(* Logix 5000 AddOnInstructionDefinition export EH_Promass10_IOL; software revision 38.00 *)

TYPE EH_CommAOI_Data :
STRUCT
   Device_Comm_Error : BOOL;
   CommSuccess : BOOL;
   CommFailed : BOOL;
   CommTimeOut : BOOL;
   StateDone : BOOL;
   NewState : BOOL;
   OldState : SINT;
   PortSize : SINT;
   DevicePort : SINT;
   MaxState : SINT;
   State : SINT;
   VendorID : INT;
   DeviceID : DINT;
   CyclicData : INT[16];
   AcyclicData : DINT[8];
   ReplayIndex : INT;
   AOI_Diagnostic : DINT;
   ConnectionStatus : DINT;
   OutputData : INT[16];
END_STRUCT
END_TYPE

ADD_ON_INSTRUCTION EH_Promass10_IOL   (* revision 1.2, vendor Endress+Hauser *)
// Promass 10 Rev 1 IO-Link
// Revision note:
// 1.2 Added HeartbeatVerification
// 1.1 Changed the Datatype from Unsigned to Signed
// Add Disconnect check
VAR_IN_OUT
   DataToSend : INT[10]; {required}
   CommAOIBusy : DINT; {required}
   ActiveComPort : DINT; {required}
   DeviceAOISendRequest : DINT; {required}
   CommError : INT; {required}
   DeviceData : EH_CommAOI_Data; {required}
END_VAR
VAR_INPUT
   iSetSimulation : BOOL; {visible}
   iSimulationVariable : INT; {visible}
   iSimulationValue : REAL; {visible}
   iSetTotalizerPresetValue : BOOL; {visible}
   iTotalizerPresetValue : REAL; {visible}
   iTotalizer_Hold : BOOL; {visible}
   iTotalizer_ResetTotalize : BOOL; {visible}
   iTotalizer_ResetHold : BOOL; {visible}
   iTotalizer_Totalize : BOOL; {visible}
   iDeviceSearch : BOOL; {visible}
   iFlowOverride : BOOL; {visible}
   iStart_HeartbeatVerification : BOOL; {visible}
END_VAR
VAR_OUTPUT
   qVendor_ID : DINT; {access Read Only, visible}
   qDevice_ID : DINT; {access Read Only, visible}
   qMassFlow : REAL; {access Read Only, visible}
   qDensity : REAL; {access Read Only, visible}
   qTemperature : REAL; {visible}
   qTotalizer1 : REAL; {access Read Only, visible}
   qExtendedDeviceStatus : INT; {access Read Only, visible}
   qSSC1_1 : BOOL; {access Read Only, visible}
   qSSC1_2 : BOOL; {access Read Only, visible}
   qSSC2_1 : BOOL; {access Read Only, visible}
   qSSC2_2 : BOOL; {access Read Only, visible}
   qSSC3_1 : BOOL; {access Read Only, visible}
   qSSC3_2 : BOOL; {access Read Only, visible}
   qSSC4_1 : BOOL; {access Read Only, visible}
   qSSC4_2 : BOOL; {access Read Only, visible}
   qProgress : SINT; {visible}
   qVerificationID : INT; {visible}
   qPassed : BOOL; {access None, visible}
   qFailed : BOOL; {access None, visible}
   qAOI_Diagnostic : DINT; {access Read Only, visible}
END_VAR
VAR_IN_OUT
   qAOI_Diagnostic_String : STRING; {required}
END_VAR
VAR_OUTPUT
   qActual_Diagnostics_Code : DINT; {access Read Only, visible}
END_VAR
VAR_IN_OUT
   qActual_Diagnostics_String : STRING; {required}
END_VAR
VAR_OUTPUT
   qLast_Diagnostics_Code : DINT; {visible}
END_VAR
VAR_IN_OUT
   qLast_Diagnostics_String : STRING; {required}
END_VAR
VAR_OUTPUT
   qCommError : DINT; {access None}
   qCommunicationBusy : DINT; {access Read Only, visible}
   qDeviceConnectionError : BOOL; {access Read Only, visible}
END_VAR
VAR
   Calc_DID : DINT; {access None}
   Calc_VID : DINT; {access None}
   Calc_Data : DINT; {access None}
   Cond_DINT : DINT; {access None}
   Temp_DINT : DINT; {access None}
   Calc_Cond : DINT; {access None}
   Cald_Temp : DINT; {access None}
   Calc_Temp : DINT; {access None}
   Calc_CondenStatus : DINT; {access None}
   CMD_Index : INT; {access None}
   CMD_Subindex : INT; {access None}
   CMD_ByteLength : INT; {access None}
   oldCondStatus : INT; {access None}
   SetSimulation : SINT; {access None}
   SetTotalizer : SINT; {access None}
   oldSetSimulation : SINT; {access None}
   oldSetTotalizer : SINT; {access None}
   Trigger : BOOL; {access None}
   CMD_Rd : BOOL; {access None}
   CMD_Wr : BOOL; {access None}
   SimulationDINT : DINT; {access None}
   SimulationReal : DINT; {access None}
   Calc_Out : DINT; {access None}
   Calc_Level : DINT; {access None}
   Calc_Pressure : DINT; {access None}
   Pressure_DINT : DINT; {access None}
   Level_DINT : DINT; {access None}
   InputByteLength : DINT; {access None}
   AOI_Prio : BOOL; {access None}
   ActiveAOI : BOOL; {access None}
   StateMin : DINT; {access None}
   firstTimeDone : BOOL; {access None}
   Calc_Connection_Status : DINT; {access None}
   NextStep : BOOL; {access None}
   OldStatus : DINT; {access None}
   ChangedStatus : BOOL; {access None}
   CondStatusChanged : BOOL; {access None}
   Calc_MassFlow : DINT; {access None}
   Calc_Density : DINT; {access None}
   Calc_Temperature : DINT; {access None}
   Calc_Totalizer1 : DINT; {access None}
   Calc_ExtendedDeviceStatus : DINT; {access None}
   MassFlow_DINT : DINT; {access None}
   Density_DINT : DINT; {access None}
   Totalizer1_DINT : DINT; {access None}
   SimChanged : BOOL; {access None}
   TotChanged : BOOL; {access None}
   Skip : BOOL; {access None}
   CondStatusActive : BOOL; {access None}
   SimActive : BOOL; {access None}
   TotActive : BOOL; {access None}
   DeviceID : DINT; {access None}
   FALSE : BOOL; {access None}
   TRUE : BOOL := 1; {access None}
   temp_string1 : STRING; {access None}
   temp_string2 : STRING; {access None}
   Start_HeartbeatVerification : SINT; {access None}
   oldStart_HeartbeatVerification : SINT; {access None}
   HeartbeatVerificationChanged : BOOL; {access None}
   HeartbeatVerificationActive : BOOL; {access None}
END_VAR

ROUTINE Logic   (* structured text *)
// Picomag Communication via AL1323
   // =======================================================================
   // Endress+Hauser Digital Solutions
   // ©Copyright (2024) All Rights Reserved
   // =======================================================================
   // Name:                EH_Promass10_IOL
   // Version:             1.2
   // Datum:               11.2025
   // Library:             01.01.00
   // Engineering:         Studio5000 V38.00.00
   // Author:              EH
   // =======================================================================
   
   qAOI_Diagnostic := DeviceData.AOI_Diagnostic;
   qCommunicationBusy := CommAOIBusy;
   DeviceID := 9728513;
   StateMin := 0;
   DeviceData.MaxState := 98;
   
   if DeviceData.DevicePort = 0 or DeviceData.DeviceID <> DeviceID or DeviceData.ConnectionStatus <> 1 then
   
   	qVendor_ID := DeviceData.VendorID;
   	qDevice_ID := DeviceData.DeviceID;
   	qMassFlow	:= 0;
   	qDensity	:= 0;
   	qTemperature	:= 0;
   	qTotalizer1	:= 0;
   	qExtendedDeviceStatus	:= 0;
   	qSSC1_1	:= 0;
   	qSSC1_2	:= 0;
   	qSSC2_1	:= 0;
   	qSSC2_2	:= 0;
   	qSSC3_1	:= 0;
   	qSSC3_2	:= 0;
   	qSSC4_1	:= 0;
   	qSSC4_2	:= 0;
   	qActual_Diagnostics_Code	:= 0;
   	qLast_Diagnostics_Code	:= 0;
   	qLast_Diagnostics_String	:= '';
   	qPassed := FALSE;
   	qFailed := FALSE;
   	oldCondStatus := 0;
   	CondStatusChanged := FALSE;
   
   	if DeviceData.DevicePort = 0 then
   
   		qActual_Diagnostics_String	:= 'Device Port is Zero';
   		DeviceData.AOI_Diagnostic.1 := TRUE;
   
   	elsif DeviceData.ConnectionStatus <> 1 then
   
   		qActual_Diagnostics_String	:= 'No Device connected';
   		qDeviceConnectionError := TRUE;
   
   	elsif DeviceData.DeviceID <> DeviceID then
   
   		qActual_Diagnostics_String	:= 'Wrong DeviceID';
   		DeviceData.AOI_Diagnostic.2 := TRUE;
   	end_if;
   
   else
   
   	if qActual_Diagnostics_Code = 0  then
   
   		qActual_Diagnostics_String	:= '--------';
   
   	end_if;
   
   	if qLast_Diagnostics_Code = 0 then
   
   		qLast_Diagnostics_String	:= '--------';
   
   	end_if;
   
   	DeviceData.AOI_Diagnostic.1 := FALSE;
   	qDeviceConnectionError := FALSE;
   	DeviceData.AOI_Diagnostic.2  := FALSE;
   
   end_if;
   
   // Case device disconnected during communication to avoid blocking the communication
   if (DeviceData.AOI_Diagnostic.0 or qDeviceConnectionError or DeviceData.AOI_Diagnostic.2) and ActiveAOI and ActiveComPort = DeviceData.DevicePort and CommAOIBusy = 1 then
   
   	DeviceData.State := 0;
   	CommAOIBusy := 0;
   	DeviceAOISendRequest.[DeviceData.DevicePort] := 0;
   	ActiveComPort := 0;
   	ActiveAOI := 0;
   	DataToSend[0] := 0;
   	DataToSend[1] := 0;
   	DataToSend[2] := 0;
   	DataToSend[3] := 0;
   	DataToSend[4] := 0;
   	DataToSend[5] := 0;
   	DataToSend[6] := 0;
   	DataToSend[7] := 0;
   	DataToSend[8] := 0;
   	DataToSend[9] := 0;
   	DeviceData.StateDone := FALSE;
   	DeviceData.NewState := FALSE;
   	DeviceData.OldState := 0;
   	ActiveAOI := FALSE;
   
   end_if;
   
   if not DeviceData.AOI_Diagnostic.0
   	and not qDeviceConnectionError
   	and not DeviceData.AOI_Diagnostic.2
   	and DeviceData.DevicePort > 0 then
   
   	//*********************************
   	//Vendor ID
   	//*********************************
   
   		qVendor_ID := DeviceData.VendorID;
   
   	//*********************************
   	//Device ID
   	//*********************************
   
   		qDevice_ID := DeviceData.DeviceID;
   
   	//*********************************
   	// Promag 10 Cyclic Input
   	//*********************************
   
   		Calc_MassFlow				:= 0;
   		Calc_Density				:= 2;
   		Calc_Temperature			:= 4;
   		Calc_Totalizer1				:= 6;
   		Calc_ExtendedDeviceStatus	:= 8;
   
   	//*********************************
   	//Process Data MassFlow
   	//*********************************
   
   		Temp_DINT	 := DeviceData.CyclicData[Calc_MassFlow+1];
   		Temp_DINT.8	 := DeviceData.CyclicData[Calc_MassFlow+1].8;
   		Temp_DINT.9  := DeviceData.CyclicData[Calc_MassFlow+1].9;
   		Temp_DINT.10 := DeviceData.CyclicData[Calc_MassFlow+1].10;
   		Temp_DINT.11 := DeviceData.CyclicData[Calc_MassFlow+1].11;
   		Temp_DINT.12 := DeviceData.CyclicData[Calc_MassFlow+1].12;
   		Temp_DINT.13 := DeviceData.CyclicData[Calc_MassFlow+1].13;
   		Temp_DINT.14 := DeviceData.CyclicData[Calc_MassFlow+1].14;
   		Temp_DINT.15 := DeviceData.CyclicData[Calc_MassFlow+1].15;
   		Temp_DINT.16 := DeviceData.CyclicData[Calc_MassFlow].0;
   		Temp_DINT.17 := DeviceData.CyclicData[Calc_MassFlow].1;
   		Temp_DINT.18 := DeviceData.CyclicData[Calc_MassFlow].2;
   		Temp_DINT.19 := DeviceData.CyclicData[Calc_MassFlow].3;
   		Temp_DINT.20 := DeviceData.CyclicData[Calc_MassFlow].4;
   		Temp_DINT.21 := DeviceData.CyclicData[Calc_MassFlow].5;
   		Temp_DINT.22 := DeviceData.CyclicData[Calc_MassFlow].6;
   		Temp_DINT.23 := DeviceData.CyclicData[Calc_MassFlow].7;
   		Temp_DINT.24 := DeviceData.CyclicData[Calc_MassFlow].8;
   		Temp_DINT.25 := DeviceData.CyclicData[Calc_MassFlow].9;
   		Temp_DINT.26 := DeviceData.CyclicData[Calc_MassFlow].10;
   		Temp_DINT.27 := DeviceData.CyclicData[Calc_MassFlow].11;
   		Temp_DINT.28 := DeviceData.CyclicData[Calc_MassFlow].12;
   		Temp_DINT.29 := DeviceData.CyclicData[Calc_MassFlow].13;
   		Temp_DINT.30 := DeviceData.CyclicData[Calc_MassFlow].14;
   		Temp_DINT.31 := DeviceData.CyclicData[Calc_MassFlow].15;
   
   		COP(Temp_DINT,qMassFlow,1);
   
   	//*********************************
   	//Process Data Density
   	//*********************************
   
   		Temp_DINT	 := DeviceData.CyclicData[Calc_Density+1];
   		Temp_DINT.8	 := DeviceData.CyclicData[Calc_Density+1].8;
   		Temp_DINT.9	 := DeviceData.CyclicData[Calc_Density+1].9;
   		Temp_DINT.10 := DeviceData.CyclicData[Calc_Density+1].10;
   		Temp_DINT.11 := DeviceData.CyclicData[Calc_Density+1].11;
   		Temp_DINT.12 := DeviceData.CyclicData[Calc_Density+1].12;
   		Temp_DINT.13 := DeviceData.CyclicData[Calc_Density+1].13;
   		Temp_DINT.14 := DeviceData.CyclicData[Calc_Density+1].14;
   		Temp_DINT.15 := DeviceData.CyclicData[Calc_Density+1].15;
   		Temp_DINT.16 := DeviceData.CyclicData[Calc_Density].0;
   		Temp_DINT.17 := DeviceData.CyclicData[Calc_Density].1;
   		Temp_DINT.18 := DeviceData.CyclicData[Calc_Density].2;
   		Temp_DINT.19 := DeviceData.CyclicData[Calc_Density].3;
   		Temp_DINT.20 := DeviceData.CyclicData[Calc_Density].4;
   		Temp_DINT.21 := DeviceData.CyclicData[Calc_Density].5;
   		Temp_DINT.22 := DeviceData.CyclicData[Calc_Density].6;
   		Temp_DINT.23 := DeviceData.CyclicData[Calc_Density].7;
   		Temp_DINT.24 := DeviceData.CyclicData[Calc_Density].8;
   		Temp_DINT.25 := DeviceData.CyclicData[Calc_Density].9;
   		Temp_DINT.26 := DeviceData.CyclicData[Calc_Density].10;
   		Temp_DINT.27 := DeviceData.CyclicData[Calc_Density].11;
   		Temp_DINT.28 := DeviceData.CyclicData[Calc_Density].12;
   		Temp_DINT.29 := DeviceData.CyclicData[Calc_Density].13;
   		Temp_DINT.30 := DeviceData.CyclicData[Calc_Density].14;
   		Temp_DINT.31 := DeviceData.CyclicData[Calc_Density].15;
   
   		COP(Temp_DINT,qDensity,1);
   
   	//*********************************
   	// Process Parameter Temperature
   	//*********************************
   
   		Temp_DINT	 := DeviceData.CyclicData[Calc_Temperature+1];
   		Temp_DINT.8	 := DeviceData.CyclicData[Calc_Temperature+1].8;
   		Temp_DINT.9	 := DeviceData.CyclicData[Calc_Temperature+1].9;
   		Temp_DINT.10 := DeviceData.CyclicData[Calc_Temperature+1].10;
   		Temp_DINT.11 := DeviceData.CyclicData[Calc_Temperature+1].11;
   		Temp_DINT.12 := DeviceData.CyclicData[Calc_Temperature+1].12;
   		Temp_DINT.13 := DeviceData.CyclicData[Calc_Temperature+1].13;
   		Temp_DINT.14 := DeviceData.CyclicData[Calc_Temperature+1].14;
   		Temp_DINT.15 := DeviceData.CyclicData[Calc_Temperature+1].15;
   		Temp_DINT.16 := DeviceData.CyclicData[Calc_Temperature].0;
   		Temp_DINT.17 := DeviceData.CyclicData[Calc_Temperature].1;
   		Temp_DINT.18 := DeviceData.CyclicData[Calc_Temperature].2;
   		Temp_DINT.19 := DeviceData.CyclicData[Calc_Temperature].3;
   		Temp_DINT.20 := DeviceData.CyclicData[Calc_Temperature].4;
   		Temp_DINT.21 := DeviceData.CyclicData[Calc_Temperature].5;
   		Temp_DINT.22 := DeviceData.CyclicData[Calc_Temperature].6;
   		Temp_DINT.23 := DeviceData.CyclicData[Calc_Temperature].7;
   		Temp_DINT.24 := DeviceData.CyclicData[Calc_Temperature].8;
   		Temp_DINT.25 := DeviceData.CyclicData[Calc_Temperature].9;
   		Temp_DINT.26 := DeviceData.CyclicData[Calc_Temperature].10;
   		Temp_DINT.27 := DeviceData.CyclicData[Calc_Temperature].11;
   		Temp_DINT.28 := DeviceData.CyclicData[Calc_Temperature].12;
   		Temp_DINT.29 := DeviceData.CyclicData[Calc_Temperature].13;
   		Temp_DINT.30 := DeviceData.CyclicData[Calc_Temperature].14;
   		Temp_DINT.31 := DeviceData.CyclicData[Calc_Temperature].15;
   
   		COP(Temp_DINT,qTemperature,1);
   
   	//*********************************
   	// Process Parameter Totalizer1
   	//*********************************
   
   		Temp_DINT	 := DeviceData.CyclicData[Calc_Totalizer1+1];
   		Temp_DINT.8	 := DeviceData.CyclicData[Calc_Totalizer1+1].8;
   		Temp_DINT.9	 := DeviceData.CyclicData[Calc_Totalizer1+1].9;
   		Temp_DINT.10 := DeviceData.CyclicData[Calc_Totalizer1+1].10;
   		Temp_DINT.11 := DeviceData.CyclicData[Calc_Totalizer1+1].11;
   		Temp_DINT.12 := DeviceData.CyclicData[Calc_Totalizer1+1].12;
   		Temp_DINT.13 := DeviceData.CyclicData[Calc_Totalizer1+1].13;
   		Temp_DINT.14 := DeviceData.CyclicData[Calc_Totalizer1+1].14;
   		Temp_DINT.15 := DeviceData.CyclicData[Calc_Totalizer1+1].15;
   		Temp_DINT.16 := DeviceData.CyclicData[Calc_Totalizer1].0;
   		Temp_DINT.17 := DeviceData.CyclicData[Calc_Totalizer1].1;
   		Temp_DINT.18 := DeviceData.CyclicData[Calc_Totalizer1].2;
   		Temp_DINT.19 := DeviceData.CyclicData[Calc_Totalizer1].3;
   		Temp_DINT.20 := DeviceData.CyclicData[Calc_Totalizer1].4;
   		Temp_DINT.21 := DeviceData.CyclicData[Calc_Totalizer1].5;
   		Temp_DINT.22 := DeviceData.CyclicData[Calc_Totalizer1].6;
   		Temp_DINT.23 := DeviceData.CyclicData[Calc_Totalizer1].7;
   		Temp_DINT.24 := DeviceData.CyclicData[Calc_Totalizer1].8;
   		Temp_DINT.25 := DeviceData.CyclicData[Calc_Totalizer1].9;
   		Temp_DINT.26 := DeviceData.CyclicData[Calc_Totalizer1].10;
   		Temp_DINT.27 := DeviceData.CyclicData[Calc_Totalizer1].11;
   		Temp_DINT.28 := DeviceData.CyclicData[Calc_Totalizer1].12;
   		Temp_DINT.29 := DeviceData.CyclicData[Calc_Totalizer1].13;
   		Temp_DINT.30 := DeviceData.CyclicData[Calc_Totalizer1].14;
   		Temp_DINT.31 := DeviceData.CyclicData[Calc_Totalizer1].15;
   
   		COP(Temp_DINT,qTotalizer1,1);
   
   	//*********************************
   	// Extended device Status
   	//*********************************
   
   		qExtendedDeviceStatus.0 := DeviceData.CyclicData[Calc_ExtendedDeviceStatus].8;
   		qExtendedDeviceStatus.1 := DeviceData.CyclicData[Calc_ExtendedDeviceStatus].9;
   		qExtendedDeviceStatus.2 := DeviceData.CyclicData[Calc_ExtendedDeviceStatus].10;
   		qExtendedDeviceStatus.3 := DeviceData.CyclicData[Calc_ExtendedDeviceStatus].11;
   		qExtendedDeviceStatus.4 := DeviceData.CyclicData[Calc_ExtendedDeviceStatus].12;
   		qExtendedDeviceStatus.5 := DeviceData.CyclicData[Calc_ExtendedDeviceStatus].13;
   		qExtendedDeviceStatus.6 := DeviceData.CyclicData[Calc_ExtendedDeviceStatus].14;
   		qExtendedDeviceStatus.7 := DeviceData.CyclicData[Calc_ExtendedDeviceStatus].15;
   
   	//*********************************
   	// Process Parameter SSC
   	//*********************************
   
   		qSSC1_1 := DeviceData.CyclicData[Calc_ExtendedDeviceStatus].0;
   		qSSC1_2 := DeviceData.CyclicData[Calc_ExtendedDeviceStatus].1;
   
   		qSSC2_1 := DeviceData.CyclicData[Calc_ExtendedDeviceStatus].2;
   		qSSC2_2 := DeviceData.CyclicData[Calc_ExtendedDeviceStatus].3;
   
   		qSSC3_1 := DeviceData.CyclicData[Calc_ExtendedDeviceStatus].4;
   		qSSC3_2 := DeviceData.CyclicData[Calc_ExtendedDeviceStatus].5;
   
   		qSSC4_1 := DeviceData.CyclicData[Calc_ExtendedDeviceStatus].6;
   		qSSC4_2 := DeviceData.CyclicData[Calc_ExtendedDeviceStatus].7;
   
   	//*********************************
   	// Process Output Parameter
   	//*********************************
   
   		DeviceData.OutputData[0].4 := iDeviceSearch;		//Device Specific
   		DeviceData.OutputData[0].5 := iFlowOverride;
   		DeviceData.OutputData[0].6 := iTotalizer_Hold;
   		DeviceData.OutputData[0].7 := iTotalizer_ResetTotalize;
   		DeviceData.OutputData[0].8 := iTotalizer_ResetHold;
   		DeviceData.OutputData[0].9 := iTotalizer_Totalize;
   
   	//*********************************
   	// Checking for Changed Status @ Input or Condenced Status
   	//*********************************
   
   	SetSimulation.0 := iSetSimulation;
   	SetTotalizer.0 := iSetTotalizerPresetValue;
   	Start_HeartbeatVerification.0 := iStart_HeartbeatVerification;
   
   	if oldCondStatus <> qExtendedDeviceStatus and not CondStatusChanged then
   
   		CondStatusChanged := TRUE;
   		oldCondStatus := qExtendedDeviceStatus;
   
   	end_if;
   
   	if oldSetSimulation <> SetSimulation and not SimChanged then
   
   		if oldSetSimulation < SetSimulation then
   
   			SimChanged := TRUE;
   
   		end_if;
   
   		oldSetSimulation := SetSimulation;
   
   	end_if;
   
   	if oldSetTotalizer <> SetTotalizer and not TotChanged then
   
   		if oldSetTotalizer < SetTotalizer then
   
   			TotChanged := TRUE;
   
   		end_if;
   
   		oldSetTotalizer := SetTotalizer;
   
   	end_if;
   
   	if oldStart_HeartbeatVerification <> Start_HeartbeatVerification and not HeartbeatVerificationChanged then
   
   		if oldStart_HeartbeatVerification < Start_HeartbeatVerification then
   
   			HeartbeatVerificationChanged := TRUE;
   
   		end_if;
   
   		oldStart_HeartbeatVerification := Start_HeartbeatVerification;
   
   	end_if;
   
   	if CondStatusChanged
   	and not ActiveAOI
   	and not CondStatusActive
   	and not Skip then
   
   		DeviceAOISendRequest.[DeviceData.DevicePort] := TRUE;
   		CondStatusActive := TRUE;
   		Skip := TRUE;
   
   	elsif SimChanged
   		and not ActiveAOI
   		and not SimActive
   		and not Skip then
   
   		DeviceAOISendRequest.[DeviceData.DevicePort] := TRUE;
   		SimActive := TRUE;
   		Skip := TRUE;
   
   	elsif TotChanged
   		and not ActiveAOI
   		and not TotActive
   		and not Skip then
   
   		DeviceAOISendRequest.[DeviceData.DevicePort] := TRUE;
   		TotActive := TRUE;
   		Skip := TRUE;
   
   	elsif HeartbeatVerificationChanged
   		and not ActiveAOI
   		and not HeartbeatVerificationActive
   		and not Skip then
   
   		DeviceAOISendRequest.[DeviceData.DevicePort] := TRUE;
   		HeartbeatVerificationActive := TRUE;
   		Skip := TRUE;
   
   	end_if;
   
   	if ActiveComPort = DeviceData.DevicePort then
   
   		AOI_Prio := TRUE;
   
   	else
   
   		AOI_Prio := FALSE;
   
   	end_if;
   
   	if (SimActive or TotActive or HeartbeatVerificationActive or CondStatusActive) and CommAOIBusy = 1  and DeviceData.State = 0 and AOI_Prio and not ActiveAOI then
   
   		ActiveAOI := TRUE;
   		Skip := FALSE;
   
   	end_if;
   
   	qCommunicationBusy := CommAOIBusy;
   	qAOI_Diagnostic :=DeviceData.AOI_Diagnostic;
   
   	//*********************************
   	// States for Execution
   	//*********************************
   
   	if ActiveAOI or DeviceData.State = DeviceData.MaxState then
   
   	case DeviceData.State of
   
   		//*********************************
   		0: // Start
   		//*********************************
   
   			Trigger := FALSE;
   			CMD_Index := 0;
   			CMD_Subindex := 0;
   			CMD_Wr := FALSE;
   			CMD_Rd := FALSE;
   			CMD_ByteLength := 0;
   
   			if DeviceData.DevicePort = ActiveComPort then
   
   				DeviceData.CommSuccess := FALSE;
   				DeviceData.CommTimeOut := FALSE;
   				DeviceData.NewState := TRUE;
   				DeviceData.StateDone := FALSE;
   
   			end_if;
   
   			if SimActive then
   
   				DeviceData.AOI_Diagnostic := 0;
   				DeviceData.State := 1;
   
   			elsif TotActive then
   				DeviceData.AOI_Diagnostic := 0;
   				DeviceData.State := 20;
   
   			elsif HeartbeatVerificationActive then
   
   				DeviceData.AOI_Diagnostic := 0;
   				DeviceData.State := 80;
   
   			elsif CondStatusChanged then
   
   				DeviceData.State := 90;
   
   			end_if;
   
   	//*********************************
   	1: // Set Simulation Variable
   	//*********************************
   
   			CMD_Index := 2066;
   			CMD_Subindex := 0;
   			CMD_Wr := TRUE;	// Only Read or Write can be active
   			CMD_Rd := FALSE;
   			CMD_ByteLength := 2;	//Check Length
   			DataToSend[6]:= 0;
   			DataToSend[7]:= 0;
   
   			// 0 = Off, 1 = Mass flow, 2 = Volume flow, 3 = Corrected volume flow, 4 = Density, 7 = Temperature
   			if iSimulationVariable > 0 then
   
   				DataToSend[6].8 := iSimulationVariable.0;
   				DataToSend[6].9 := iSimulationVariable.1;
   				DataToSend[6].10 := iSimulationVariable.2;
   				DataToSend[6].11 := iSimulationVariable.3;
   				DataToSend[6].12 := iSimulationVariable.4;
   				DataToSend[6].13 := iSimulationVariable.5;
   				DataToSend[6].14 := iSimulationVariable.6;
   				DataToSend[6].15 := iSimulationVariable.7;
   
   			else
   
   				DataToSend[6] := 0;
   				DataToSend[7] := 0;
   
   			end_if;
   
   			Trigger := TRUE;
   
   			if DeviceData.NewState then
   
   				DeviceData.StateDone := TRUE;
   
   			end_if;
   
   			if  DeviceData.CommSuccess and DeviceData.ReplayIndex = CMD_Index then
   
   				Trigger := FALSE;
   				DeviceData.OldState := DeviceData.State;
   				DeviceData.State := DeviceData.State + 1;
   				DeviceData.CommSuccess := FALSE;
   				DeviceData.AcyclicData[0] := 0;
   				DeviceData.NewState := TRUE;
   
   			elsif DeviceData.CommTimeOut then
   
   				temp_string1 := 'Error in step ';
   				Temp_DINT := DeviceData.State;
   				DTOS(Temp_DINT, temp_string2);
   				CONCAT(temp_string1, temp_string2, qAOI_Diagnostic_String);
   
   				DeviceData.OldState := DeviceData.State;
   				DeviceData.State := DeviceData.MaxState;
   				DeviceData.CommTimeOut := FALSE;
   				DeviceData.AcyclicData[0] := 0;
   				DeviceData.NewState := TRUE;
   
   			end_if;
   
   
   		//*********************************
   		2: // Set Simulation Value
   		//*********************************
   
   			CMD_Index := 2124;
   			CMD_Subindex := 0;
   			CMD_Wr := TRUE;
   			CMD_Rd := FALSE;
   			CMD_ByteLength := 4;
   			DataToSend[6]:= 0;
   			DataToSend[7]:= 0;
   
   		 	COP(iSimulationValue,SimulationDINT,1);		// Copy the Bits from the Real in a DINT
   
   			DataToSend[6].0 :=  SimulationDINT.24;
   			DataToSend[6].1 :=  SimulationDINT.25;
   			DataToSend[6].2 :=  SimulationDINT.26;
   			DataToSend[6].3 :=  SimulationDINT.27;
   			DataToSend[6].4 :=  SimulationDINT.28;
   			DataToSend[6].5 :=  SimulationDINT.29;
   			DataToSend[6].6 :=  SimulationDINT.30;
   			DataToSend[6].7 :=  SimulationDINT.31;
   			DataToSend[6].8 :=  SimulationDINT.16;
   			DataToSend[6].9 :=  SimulationDINT.17;
   			DataToSend[6].10 := SimulationDINT.18;
   			DataToSend[6].11 := SimulationDINT.19;
   			DataToSend[6].12 := SimulationDINT.20;
   			DataToSend[6].13 := SimulationDINT.21;
   			DataToSend[6].14 := SimulationDINT.22;
   			DataToSend[6].15 := SimulationDINT.23;
   			DataToSend[7].0  := SimulationDINT.8;
   			DataToSend[7].1  := SimulationDINT.9;
   			DataToSend[7].2  := SimulationDINT.10;
   			DataToSend[7].3  := SimulationDINT.11;
   			DataToSend[7].4  := SimulationDINT.12;
   			DataToSend[7].5  := SimulationDINT.13;
   			DataToSend[7].6  := SimulationDINT.14;
   			DataToSend[7].7  := SimulationDINT.15;
   			DataToSend[7].8  := SimulationDINT.0;
   			DataToSend[7].9  := SimulationDINT.1;
   			DataToSend[7].10 := SimulationDINT.2;
   			DataToSend[7].11 := SimulationDINT.3;
   			DataToSend[7].12 := SimulationDINT.4;
   			DataToSend[7].13 := SimulationDINT.5;
   			DataToSend[7].14 := SimulationDINT.6;
   			DataToSend[7].15 := SimulationDINT.7;
   
   			Trigger := TRUE;
   
   			if DeviceData.NewState then
   
   				DeviceData.StateDone := TRUE;
   
   			end_if;
   
   			if DeviceData.CommSuccess and DeviceData.ReplayIndex = CMD_Index then
   
   				Trigger := FALSE;
   				DeviceData.OldState := DeviceData.State;
   				DeviceData.State := DeviceData.MaxState;
   				DeviceData.CommSuccess := FALSE;
   				DeviceData.AcyclicData[0] := 0;
   				DeviceData.NewState := TRUE;
   
   			elsif DeviceData.CommTimeOut then
   
   				temp_string1 := 'Error in step ';
   				Temp_DINT := DeviceData.State;
   				DTOS(Temp_DINT, temp_string2);
   				CONCAT(temp_string1, temp_string2, qAOI_Diagnostic_String);
   
   				DeviceData.OldState := DeviceData.State;
   				DeviceData.State := DeviceData.MaxState;	//Check State
   				DeviceData.CommTimeOut := FALSE;
   				DeviceData.AcyclicData[0] := 0;
   				DeviceData.NewState := TRUE;
   
   			end_if;
   
   		//*********************************
   		20: // Totalizer 1 Preset value
   		//*********************************
   
   			CMD_Index := 2103;
   			CMD_Subindex := 0;
   			CMD_Wr := TRUE;								// Only Read or Write can be active = 1
   			CMD_Rd := FALSE;
   			CMD_ByteLength := 4;
   			DataToSend[6]:= 0;
   			DataToSend[7]:= 0;
   
   		 	COP(iTotalizerPresetValue,SimulationDINT,1); // Copy the Bits from the Real in a DINT
   
   			DataToSend[6].0 :=  SimulationDINT.24;
   			DataToSend[6].1 :=  SimulationDINT.25;
   			DataToSend[6].2 :=  SimulationDINT.26;
   			DataToSend[6].3 :=  SimulationDINT.27;
   			DataToSend[6].4 :=  SimulationDINT.28;
   			DataToSend[6].5 :=  SimulationDINT.29;
   			DataToSend[6].6 :=  SimulationDINT.30;
   			DataToSend[6].7 :=  SimulationDINT.31;
   			DataToSend[6].8 :=  SimulationDINT.16;
   			DataToSend[6].9 :=  SimulationDINT.17;
   			DataToSend[6].10 := SimulationDINT.18;
   			DataToSend[6].11 := SimulationDINT.19;
   			DataToSend[6].12 := SimulationDINT.20;
   			DataToSend[6].13 := SimulationDINT.21;
   			DataToSend[6].14 := SimulationDINT.22;
   			DataToSend[6].15 := SimulationDINT.23;
   			DataToSend[7].0  := SimulationDINT.8;
   			DataToSend[7].1  := SimulationDINT.9;
   			DataToSend[7].2  := SimulationDINT.10;
   			DataToSend[7].3  := SimulationDINT.11;
   			DataToSend[7].4  := SimulationDINT.12;
   			DataToSend[7].5  := SimulationDINT.13;
   			DataToSend[7].6  := SimulationDINT.14;
   			DataToSend[7].7  := SimulationDINT.15;
   			DataToSend[7].8  := SimulationDINT.0;
   			DataToSend[7].9  := SimulationDINT.1;
   			DataToSend[7].10 := SimulationDINT.2;
   			DataToSend[7].11 := SimulationDINT.3;
   			DataToSend[7].12 := SimulationDINT.4;
   			DataToSend[7].13 := SimulationDINT.5;
   			DataToSend[7].14 := SimulationDINT.6;
   			DataToSend[7].15 := SimulationDINT.7;
   
   			Trigger := TRUE;
   
   			if DeviceData.NewState then
   				DeviceData.StateDone := TRUE;
   			end_if;
   
   			if  DeviceData.CommSuccess and DeviceData.ReplayIndex = CMD_Index then
   
   				Trigger := FALSE;
   				DeviceData.OldState := DeviceData.State;
   				DeviceData.State := DeviceData.State + 1;
   				DeviceData.CommSuccess := FALSE;
   				DeviceData.AcyclicData[0] := 0;
   				DeviceData.NewState := TRUE;
   
   			 elsif DeviceData.CommTimeOut then
   
   				temp_string1 := 'Error in step ';
   				Temp_DINT := DeviceData.State;
   				DTOS(Temp_DINT, temp_string2);
   				CONCAT(temp_string1, temp_string2, qAOI_Diagnostic_String);
   
   				DeviceData.OldState := DeviceData.State;
   				DeviceData.State := DeviceData.MaxState;	//Check State
   				DeviceData.CommTimeOut := FALSE;
   				DeviceData.AcyclicData[0] := 0;
   				DeviceData.NewState := TRUE;
   
   			end_if;
   
   		//*********************************
   		21: // Totalizer 1 Control
   		//*********************************
   
   			CMD_Index := 2100;
   			CMD_Subindex := 0;
   			CMD_Wr := TRUE;
   			CMD_Rd := FALSE;
   			CMD_ByteLength := 2;
   			DataToSend[6]:= 0;
   			DataToSend[7]:= 0;
   
   			DataToSend[6].9:= 1; // Preset + hold
   
   			Trigger := TRUE;
   
   			if DeviceData.NewState then
   
   				DeviceData.StateDone := TRUE;
   
   			end_if;
   
   			if  DeviceData.CommSuccess and DeviceData.ReplayIndex = CMD_Index then
   
   				Trigger := FALSE;
   				DeviceData.OldState := DeviceData.State;
   				DeviceData.State := DeviceData.MaxState;
   				DeviceData.CommSuccess := FALSE;
   				DeviceData.AcyclicData[0] := 0;
   				DeviceData.NewState := TRUE;
   
   			elsif DeviceData.CommTimeOut then
   
   				temp_string1 := 'Error in step ';
   				Temp_DINT := DeviceData.State;
   				DTOS(Temp_DINT, temp_string2);
   				CONCAT(temp_string1, temp_string2, qAOI_Diagnostic_String);
   
   				DeviceData.OldState := DeviceData.State;
   				DeviceData.State := DeviceData.MaxState;
   				DeviceData.CommTimeOut := FALSE;
   				DeviceData.AcyclicData[0] := 0;
   				DeviceData.NewState := TRUE;
   
   			end_if;
   
   		//*********************************
   		80: // Check Heartbeat Verification activation
   		//*********************************
   
   			CMD_Index := 12342;
   			CMD_Subindex := 0;
   			CMD_Wr := FALSE;
   			CMD_Rd := TRUE;
   			CMD_ByteLength := 1;
   			Trigger := TRUE;
   			DataToSend[6]:= 0;
   			DataToSend[7]:= 0;
   
   			if DeviceData.NewState then
   
   				DeviceData.StateDone := TRUE;
   
   			end_if;
   
   			if  DeviceData.CommSuccess and DeviceData.ReplayIndex = CMD_Index then
   
   				if DeviceData.AcyclicData[0] = 1 then
   
   					DeviceData.State := DeviceData.State + 1;
   
   				else
   					qAOI_Diagnostic_String := 'Step 80: Software Option not activated ';
   
   					DeviceData.OldState := DeviceData.State;
   					DeviceData.State := DeviceData.MaxState;
   
   				end_if;
   
   				Trigger := FALSE;
   				DeviceData.CommSuccess := FALSE;
   				DeviceData.AcyclicData[0] := 0;
   				DeviceData.NewState := TRUE;
   
   			 elsif DeviceData.CommTimeOut then
   
   				temp_string1 := 'Error in step ';
   				Temp_DINT := DeviceData.State;
   				DTOS(Temp_DINT, temp_string2);
   				CONCAT(temp_string1, temp_string2, qAOI_Diagnostic_String);
   
   				DeviceData.OldState := DeviceData.State;
   				DeviceData.State := DeviceData.MaxState;
   				DeviceData.CommTimeOut := FALSE;
   				DeviceData.AcyclicData[0] := 0;
   				DeviceData.NewState := TRUE;
   
   			end_if;
   
   		//*********************************
   		81: // Check if Verifivation is ongoing
   		//*********************************
   
   			CMD_Index := 12323;
   			CMD_Subindex := 0;
   			CMD_Wr := FALSE;
   			CMD_Rd := TRUE;
   			CMD_ByteLength := 2;
   			Trigger := TRUE;
   
   			if DeviceData.NewState then
   
   				DeviceData.StateDone := TRUE;
   
   			end_if;
   
   			if  DeviceData.CommSuccess and DeviceData.ReplayIndex = CMD_Index then
   
   				if DeviceData.AcyclicData[0] <> 8 then
   
   					DeviceData.State := DeviceData.State + 1;
   
   				else
   					qAOI_Diagnostic_String := 'Step 81: Heartbeat Verification already in progress ';
   					DeviceData.OldState := DeviceData.State;
   					DeviceData.State := DeviceData.MaxState;
   					DeviceData.CommTimeOut := FALSE;
   
   				end_if;
   
   				Trigger := FALSE;
   				DeviceData.CommSuccess := FALSE;
   				DeviceData.AcyclicData[0] := 0;
   				DeviceData.NewState := TRUE;
   
   			 elsif DeviceData.CommTimeOut then
   
   				temp_string1 := 'Error in step ';
   				Temp_DINT := DeviceData.State;
   				DTOS(Temp_DINT, temp_string2);
   				CONCAT(temp_string1, temp_string2, qAOI_Diagnostic_String);
   
   				DeviceData.OldState := DeviceData.State;
   				DeviceData.State := DeviceData.MaxState;
   				DeviceData.CommTimeOut := FALSE;
   				DeviceData.AcyclicData[0] := 0;
   				DeviceData.NewState := TRUE;
   
   			end_if;
   
   		//*********************************
   		82: // Start Verification
   		//*********************************
   
   			CMD_Index := 12325;
   			CMD_Subindex := 0;
   			CMD_Wr := TRUE;
   			CMD_Rd := FALSE;
   			CMD_ByteLength := 2;
   			Trigger := TRUE;
   			DataToSend[6] := 0;
   			DataToSend[7] := 0;
   
   			DataToSend[6].8 := TRUE;
   
   			if DeviceData.NewState then
   
   				DeviceData.StateDone := TRUE;
   
   			end_if;
   
   		if DeviceData.CommSuccess and DeviceData.ReplayIndex = CMD_Index then
   
   		    Trigger := FALSE;
   		    DeviceData.CommSuccess := FALSE;
   		    DeviceData.State := DeviceData.State + 2;
   			DeviceData.AcyclicData[0] := 0;
   			DeviceData.NewState := TRUE;
   
   		elsif DeviceData.CommTimeOut then
   
   		    temp_string1 := 'Error in step ';
   		    Temp_DINT := DeviceData.State;
   		    DTOS(Temp_DINT, temp_string2);
   		    CONCAT(temp_string1, temp_string2, qAOI_Diagnostic_String);
   
   		    DeviceData.OldState := DeviceData.State;
   		    DeviceData.State := DeviceData.MaxState;
   		    DeviceData.CommTimeOut := FALSE;
   			DeviceData.AcyclicData[0] := 0;
   			DeviceData.NewState := TRUE;
   
   		end_if;
   
   
   		//*********************************
   		83: // Intermediate state
   		//*********************************
   
   			CMD_Index := 36;
   			CMD_Subindex := 0;
   			CMD_Wr := FALSE;
   			CMD_Rd := TRUE;
   			CMD_ByteLength := 1;
   			Trigger := TRUE;
   
   			if DeviceData.NewState then
   
   				DeviceData.StateDone := TRUE;
   
   			end_if;
   
   			if DeviceData.CommSuccess and DeviceData.ReplayIndex = CMD_Index then
   
   			    DeviceData.State := DeviceData.State + 1;
   			    Trigger := FALSE;
   			    DeviceData.CommSuccess := FALSE;
   				DeviceData.AcyclicData[0] := 0;
   				DeviceData.NewState := TRUE;
   
   			elsif DeviceData.CommTimeOut then
   
   			    temp_string1 := 'Error in step ';
   			    Temp_DINT := DeviceData.State;
   			    DTOS(Temp_DINT, temp_string2);
   			    CONCAT(temp_string1, temp_string2, qAOI_Diagnostic_String);
   
   			    DeviceData.OldState := DeviceData.State;
   			    DeviceData.State := DeviceData.MaxState;
   			    DeviceData.CommTimeOut := FALSE;
   				DeviceData.AcyclicData[0] := 0;
   				DeviceData.NewState := TRUE;
   
   			end_if;
   
   		//*********************************
   		84: // Read progress
   		//*********************************
   
   			CMD_Index := 2155;
   			CMD_Subindex := 0;
   			CMD_Wr := FALSE;
   			CMD_Rd := TRUE;
   			CMD_ByteLength := 1;
   			Trigger := TRUE;
   
   			if DeviceData.NewState then
   
   				DeviceData.StateDone := TRUE;
   
   			end_if;
   
   			if DeviceData.CommSuccess and DeviceData.ReplayIndex = CMD_Index then
   
   				qProgress := DeviceData.AcyclicData[0];
   
   				if DeviceData.AcyclicData[0] = 100 then
   
   					DeviceData.State := DeviceData.State + 1;
   
   				elsif DeviceData.AcyclicData[0] < 100 then
   
   					DeviceData.State := DeviceData.State - 1;
   
   				end_if;
   
   				Trigger := FALSE;
   				DeviceData.CommSuccess := FALSE;
   				DeviceData.AcyclicData[0] := 0;
   				DeviceData.NewState := TRUE;
   
   			elsif DeviceData.CommTimeOut then
   
   			    temp_string1 := 'Error in step ';
   			    Temp_DINT := DeviceData.State;
   			    DTOS(Temp_DINT, temp_string2);
   			    CONCAT(temp_string1, temp_string2, qAOI_Diagnostic_String);
   
   			    DeviceData.OldState := DeviceData.State;
   			    DeviceData.State := DeviceData.MaxState;
   			    DeviceData.CommTimeOut := FALSE;
   				DeviceData.AcyclicData[0] := 0;
   				DeviceData.NewState := TRUE;
   
   			end_if;
   
   		//*********************************
   		85: // Read status
   		//*********************************
   
   			CMD_Index := 12323;
   			CMD_Subindex := 0;
   			CMD_Wr := FALSE;
   			CMD_Rd := TRUE;
   			CMD_ByteLength := 2;
   			Trigger := TRUE;
   
   			if DeviceData.NewState then
   
   				DeviceData.StateDone := TRUE;
   
   			end_if;
   
   			if DeviceData.CommSuccess and DeviceData.ReplayIndex = CMD_Index then
   
   			    if DeviceData.AcyclicData[0] = 1 then
   
   			        DeviceData.State := DeviceData.State + 1;
   
   			    else
   			        qAOI_Diagnostic_String := 'Step 85: Heartbeat Verification not done';
   			        DeviceData.OldState := DeviceData.State;
   			        DeviceData.State := DeviceData.MaxState;
   			        DeviceData.CommTimeOut := FALSE;
   
   			    end_if;
   
   			    Trigger := FALSE;
   			    DeviceData.CommSuccess := FALSE;
   				DeviceData.AcyclicData[1] := 0;
   				DeviceData.NewState := TRUE;
   
   			elsif DeviceData.CommTimeOut then
   
   			    temp_string1 := 'Error in step ';
   			    Temp_DINT := DeviceData.State;
   			    DTOS(Temp_DINT, temp_string2);
   			    CONCAT(temp_string1, temp_string2, qAOI_Diagnostic_String);
   
   			    DeviceData.OldState := DeviceData.State;
   			    DeviceData.State := DeviceData.MaxState;
   			    DeviceData.CommTimeOut := FALSE;
   				DeviceData.AcyclicData[0] := 0;
   				DeviceData.NewState := TRUE;
   
   			end_if;
   
   		//*********************************
   		86: // Read overall result
   		//*********************************
   
   			CMD_Index := 12322;
   			CMD_Subindex := 0;
   			CMD_Wr := FALSE;
   			CMD_Rd := TRUE;
   			CMD_ByteLength := 2;
   			Trigger := TRUE;
   
   			if DeviceData.NewState then
   
   				DeviceData.StateDone := TRUE;
   
   			end_if;
   
   			if  DeviceData.CommSuccess and DeviceData.ReplayIndex = CMD_Index then
   
   				if DeviceData.AcyclicData[0] = 2 then
   
   					qPassed := TRUE;
   					qFailed := FALSE;
   
   				else
   
   					qPassed := FALSE;
   					qFailed := TRUE;
   
   				end_if;
   
   				Trigger := FALSE;
   				DeviceData.CommSuccess := FALSE;
   				DeviceData.State := DeviceData.State + 1;
   				DeviceData.AcyclicData[0] := 0;
   				DeviceData.NewState := TRUE;
   
   			 elsif DeviceData.CommTimeOut then
   
   				temp_string1 := 'Error in step ';
   				Temp_DINT := DeviceData.State;
   				DTOS(Temp_DINT, temp_string2);
   				CONCAT(temp_string1, temp_string2, qAOI_Diagnostic_String);
   
   				DeviceData.CommTimeOut := FALSE;
   				DeviceData.OldState := DeviceData.State;
   				DeviceData.State := DeviceData.MaxState;
   				DeviceData.AcyclicData[0] := 0;
   				DeviceData.NewState := TRUE;
   
   			end_if;
   
   		//*********************************
   		87: // Read Verification ID
   		//*********************************
   
   			CMD_Index := 12321;
   			CMD_Subindex := 0;
   			CMD_Wr := FALSE;
   			CMD_Rd := TRUE;
   			CMD_ByteLength := 2;
   			Trigger := TRUE;
   
   			if DeviceData.NewState then
   
   				DeviceData.StateDone := TRUE;
   
   			end_if;
   
   			if  DeviceData.CommSuccess and DeviceData.ReplayIndex = CMD_Index then
   
   				qVerificationID.0	:= DeviceData.AcyclicData[0].0;
   				qVerificationID.1	:= DeviceData.AcyclicData[0].1;
   				qVerificationID.2	:= DeviceData.AcyclicData[0].2;
   				qVerificationID.3	:= DeviceData.AcyclicData[0].3;
   				qVerificationID.4	:= DeviceData.AcyclicData[0].4;
   				qVerificationID.5	:= DeviceData.AcyclicData[0].5;
   				qVerificationID.6	:= DeviceData.AcyclicData[0].6;
   				qVerificationID.7	:= DeviceData.AcyclicData[0].7;
   				qVerificationID.8	:= DeviceData.AcyclicData[0].8;
   				qVerificationID.9	:= DeviceData.AcyclicData[0].9;
   				qVerificationID.10	:= DeviceData.AcyclicData[0].10;
   				qVerificationID.11	:= DeviceData.AcyclicData[0].11;
   				qVerificationID.12	:= DeviceData.AcyclicData[0].12;
   				qVerificationID.13	:= DeviceData.AcyclicData[0].13;
   				qVerificationID.14	:= DeviceData.AcyclicData[0].14;
   				qVerificationID.15	:= DeviceData.AcyclicData[0].15;
   
   				Trigger := FALSE;
   				DeviceData.CommSuccess := FALSE;
   				DeviceData.OldState := DeviceData.State;
   				DeviceData.State := DeviceData.MaxState;
   				DeviceData.NewState := TRUE;
   
   			 elsif DeviceData.CommTimeOut then
   
   				temp_string1 := 'Error in step ';
   				Temp_DINT := DeviceData.State;
   				DTOS(Temp_DINT, temp_string2);
   				CONCAT(temp_string1, temp_string2, qAOI_Diagnostic_String);
   
   				DeviceData.CommTimeOut := FALSE;
   				DeviceData.OldState := DeviceData.State;
   				DeviceData.State := DeviceData.MaxState;
   				DeviceData.NewState := TRUE;
   
   			end_if;
   
   		//*********************************
   		90: // Actual Diagnostic
   		//*********************************
   
   			CMD_Index := 297;
   			CMD_Subindex := 0;
   			CMD_Wr := FALSE;
   			CMD_Rd := TRUE;
   			CMD_ByteLength := 4;
   			Trigger := TRUE;
   
   			if DeviceData.NewState then
   
   				DeviceData.StateDone := TRUE;
   
   			end_if;
   
   			if  DeviceData.CommSuccess and DeviceData.ReplayIndex = CMD_Index then
   
   				qActual_Diagnostics_Code	:= DeviceData.AcyclicData[0];
   
   				case qActual_Diagnostics_Code of
   
   			        0:
   			            qActual_Diagnostics_String := '--------';
   			        16777296:
   			            qActual_Diagnostics_String := 'F910 Tubes not oscillating';
   			        16777312:
   			            qActual_Diagnostics_String := 'F437 Configuration incompatible';
   			        16777319:
   			            qActual_Diagnostics_String := 'F242 Firmware incompatible';
   			        16777323:
   			            qActual_Diagnostics_String := 'F252 Module incompatible';
   			        16777355:
   			            qActual_Diagnostics_String := 'F410 Data transfer failed';
   			        16777376:
   			            qActual_Diagnostics_String := 'F083 Memory content inconsistent';
   			        16777377:
   			            qActual_Diagnostics_String := 'F372 Sensor electronics (ISEM) faulty';
   			        16777415:
   			            qActual_Diagnostics_String := 'F372 Sensor electronics (ISEM) faulty';
   			        16777417:
   			            qActual_Diagnostics_String := 'F372 Sensor electronics (ISEM) faulty';
   			        16777428:
   			            qActual_Diagnostics_String := 'F372 Sensor electronics (ISEM) faulty';
   			        16777429:
   			            qActual_Diagnostics_String := 'F022 Temperature sensor defective';
   			        16777430:
   			            qActual_Diagnostics_String := 'F022 Temperature sensor defective';
   			        16777434:
   			            qActual_Diagnostics_String := 'F372 Sensor electronics (ISEM) faulty';
   			        16777435:
   			            qActual_Diagnostics_String := 'F062 Sensor connection faulty';
   			        16777436:
   			            qActual_Diagnostics_String := 'F062 Sensor connection faulty';
   			        16777447:
   			            qActual_Diagnostics_String := 'F082 Data storage inconsistent';
   			        16777491:
   			            qActual_Diagnostics_String := 'F062 Sensor connection faulty';
   			        16777492:
   			            qActual_Diagnostics_String := 'F062 Sensor connection faulty';
   			        16777497:
   			            qActual_Diagnostics_String := 'F222 Electronics drift';
   			        16777504:
   			            qActual_Diagnostics_String := 'F372 Sensor electronics (ISEM) faulty';
   			        16777547:
   			            qActual_Diagnostics_String := 'F201 Electronics faulty';
   			        16777578:
   			            qActual_Diagnostics_String := 'F270 Electronic module defective';
   			        16777582:
   			            qActual_Diagnostics_String := 'F383 Memory content';
   			        16777583:
   			            qActual_Diagnostics_String := 'F283 Memory content inconsistent';
   			        16777671:
   			            qActual_Diagnostics_String := 'F144 Measurement error too high';
   			        16777864:
   			            qActual_Diagnostics_String := 'F387 HistoROM data faulty';
   			        16777907:
   			            qActual_Diagnostics_String := 'F063 Exciter current faulty';
   			        16777920:
   			            qActual_Diagnostics_String := 'F252 Module incompatible';
   			        16777930:
   			            qActual_Diagnostics_String := 'F331 Firmware update failed in module 1';
   			        16777931:
   			            qActual_Diagnostics_String := 'F372 Sensor electronics (ISEM) faulty';
   			        16777932:
   			            qActual_Diagnostics_String := 'F372 Sensor electronics (ISEM) faulty';
   			        16777933:
   			            qActual_Diagnostics_String := 'F372 Sensor electronics (ISEM) faulty';
   			        16777935:
   			            qActual_Diagnostics_String := 'F372 Sensor electronics (ISEM) faulty';
   			        16777936:
   			            qActual_Diagnostics_String := 'F372 Sensor electronics (ISEM) faulty';
   			        16777937:
   			            qActual_Diagnostics_String := 'F373 Sensor electronics (ISEM) faulty';
   			        16778224:
   			            qActual_Diagnostics_String := 'F378 Electronic module supply voltage faulty';
   			        16778408:
   			            qActual_Diagnostics_String := 'F278 Display module defective';
   			        16778409:
   			            qActual_Diagnostics_String := 'F278 Display module defective';
   			        16778490:
   			            qActual_Diagnostics_String := 'F419 Power cycle required';
   			        16843466:
   			            qActual_Diagnostics_String := 'F331 Firmware update failed in module 2';
   			        16909002:
   			            qActual_Diagnostics_String := 'F331 Firmware update failed in module 3';
   			        33554576:
   			            qActual_Diagnostics_String := 'C484 Failure mode simulation active';
   			        33554579:
   			            qActual_Diagnostics_String := 'C485 Process variable simulation active';
   			        33554580:
   			            qActual_Diagnostics_String := 'C453 Flow override active';
   			        33554782:
   			            qActual_Diagnostics_String := 'C495 Diagnostic event simulation active';
   			        33554926:
   			            qActual_Diagnostics_String := 'C302 Device verification active';
   			        33554948:
   			            qActual_Diagnostics_String := 'C412 Processing download';
   			        67108970:
   			            qActual_Diagnostics_String := 'M438 Dataset different';
   			        67109090:
   			            qActual_Diagnostics_String := 'M311 Sensor electronics (ISEM) faulty';
   			        67109921:
   			            qActual_Diagnostics_String := 'M230 Date/time incorrect';
   			        67110029:
   			            qActual_Diagnostics_String := 'M231 Date/time not available';
   			        67110030:
   			            qActual_Diagnostics_String := 'M230 Date/time incorrect';
   			        134217873:
   			            qActual_Diagnostics_String := 'S842 Process value below limit';
   			        134217874:
   			            qActual_Diagnostics_String := 'S862 Partly filled pipe';
   			        134217921:
   			            qActual_Diagnostics_String := 'S833 Sensor electronics temperature too low';
   			        134217923:
   			            qActual_Diagnostics_String := 'S832 Sensor electronics temperature too high';
   			        134217924:
   			            qActual_Diagnostics_String := 'S912 Medium inhomogeneous';
   			        134217925:
   			            qActual_Diagnostics_String := 'S834 Process temperature too high';
   			        134217926:
   			            qActual_Diagnostics_String := 'S835 Process temperature too low';
   			        134217928:
   			            qActual_Diagnostics_String := 'S046 Sensor limit exceeded';
   			        134217930:
   			            qActual_Diagnostics_String := 'S046 Sensor limit exceeded';
   			        134217932:
   			            qActual_Diagnostics_String := 'S140 Sensor signal asymmetrical';
   			        134217933:
   			            qActual_Diagnostics_String := 'S913 Medium unsuitable';
   			        134217934:
   			            qActual_Diagnostics_String := 'S374 Sensor electronics (ISEM) faulty';
   			        134217951:
   			            qActual_Diagnostics_String := 'S912 Medium inhomogeneous';
   			        134218005:
   			            qActual_Diagnostics_String := 'S912 Medium inhomogeneous';
   			        134218082:
   			            qActual_Diagnostics_String := 'S912 Medium inhomogeneous';
   			        134218088:
   			            qActual_Diagnostics_String := 'S948 Oscillation damping too high';
   			        134218182:
   			            qActual_Diagnostics_String := 'S944 Monitoring failed';
   
   					else
   
   						qActual_Diagnostics_String := 'Error Code unknown';
   
   				end_case;
   
   			Trigger := FALSE;
   			DeviceData.OldState := DeviceData.State;
   			DeviceData.State := DeviceData.State + 1;
   			DeviceData.CommSuccess := FALSE;
   			DeviceData.AcyclicData[0] := 0;
   			DeviceData.NewState := TRUE;
   
   		elsif DeviceData.CommTimeOut then
   
   			temp_string1 := 'Error in step ';
   			Temp_DINT := DeviceData.State;
   			DTOS(Temp_DINT, temp_string2);
   			CONCAT(temp_string1, temp_string2, qAOI_Diagnostic_String);
   
   			DeviceData.OldState := DeviceData.State;
   			DeviceData.State := DeviceData.MaxState;
   			DeviceData.CommTimeOut := FALSE;
   			DeviceData.AcyclicData[0] := 0;
   			DeviceData.NewState := TRUE;
   
   		end_if;
   
   		//*********************************
   		91: // Last Diagnostic
   		//*********************************
   
   			CMD_Index := 298;
   			CMD_Subindex := 0;
   			CMD_Wr := FALSE;
   			CMD_Rd := TRUE;
   			CMD_ByteLength := 4;
   			Trigger := TRUE;
   
   			if DeviceData.NewState then
   
   				DeviceData.StateDone := TRUE;
   
   			end_if;
   
   			if DeviceData.CommSuccess and DeviceData.ReplayIndex = CMD_Index then
   
   				qLast_Diagnostics_Code	:= DeviceData.AcyclicData[0];
   
   				case qLast_Diagnostics_Code of
   					0:
   			            qLast_Diagnostics_String := '--------';
   			        16777296:
   			            qLast_Diagnostics_String := 'F910 Tubes not oscillating';
   			        16777312:
   			            qLast_Diagnostics_String := 'F437 Configuration incompatible';
   			        16777319:
   			            qLast_Diagnostics_String := 'F242 Firmware incompatible';
   			        16777323:
   			            qLast_Diagnostics_String := 'F252 Module incompatible';
   			        16777355:
   			            qLast_Diagnostics_String := 'F410 Data transfer failed';
   			        16777376:
   			            qLast_Diagnostics_String := 'F083 Memory content inconsistent';
   			        16777377:
   			            qLast_Diagnostics_String := 'F372 Sensor electronics (ISEM) faulty';
   			        16777415:
   			            qLast_Diagnostics_String := 'F372 Sensor electronics (ISEM) faulty';
   			        16777417:
   			            qLast_Diagnostics_String := 'F372 Sensor electronics (ISEM) faulty';
   			        16777428:
   			            qLast_Diagnostics_String := 'F372 Sensor electronics (ISEM) faulty';
   			        16777429:
   			            qLast_Diagnostics_String := 'F022 Temperature sensor defective';
   			        16777430:
   			            qLast_Diagnostics_String := 'F022 Temperature sensor defective';
   			        16777434:
   			            qLast_Diagnostics_String := 'F372 Sensor electronics (ISEM) faulty';
   			        16777435:
   			            qLast_Diagnostics_String := 'F062 Sensor connection faulty';
   			        16777436:
   			            qLast_Diagnostics_String := 'F062 Sensor connection faulty';
   			        16777447:
   			            qLast_Diagnostics_String := 'F082 Data storage inconsistent';
   			        16777491:
   			            qLast_Diagnostics_String := 'F062 Sensor connection faulty';
   			        16777492:
   			            qLast_Diagnostics_String := 'F062 Sensor connection faulty';
   			        16777497:
   			            qLast_Diagnostics_String := 'F222 Electronics drift';
   			        16777504:
   			            qLast_Diagnostics_String := 'F372 Sensor electronics (ISEM) faulty';
   			        16777547:
   			            qLast_Diagnostics_String := 'F201 Electronics faulty';
   			        16777578:
   			            qLast_Diagnostics_String := 'F270 Electronic module defective';
   			        16777582:
   			            qLast_Diagnostics_String := 'F383 Memory content';
   			        16777583:
   			            qLast_Diagnostics_String := 'F283 Memory content inconsistent';
   			        16777671:
   			            qLast_Diagnostics_String := 'F144 Measurement error too high';
   			        16777864:
   			            qLast_Diagnostics_String := 'F387 HistoROM data faulty';
   			        16777907:
   			            qLast_Diagnostics_String := 'F063 Exciter current faulty';
   			        16777920:
   			            qLast_Diagnostics_String := 'F252 Module incompatible';
   			        16777930:
   			            qLast_Diagnostics_String := 'F331 Firmware update failed in module 1';
   			        16777931:
   			            qLast_Diagnostics_String := 'F372 Sensor electronics (ISEM) faulty';
   			        16777932:
   			            qLast_Diagnostics_String := 'F372 Sensor electronics (ISEM) faulty';
   			        16777933:
   			            qLast_Diagnostics_String := 'F372 Sensor electronics (ISEM) faulty';
   			        16777935:
   			            qLast_Diagnostics_String := 'F372 Sensor electronics (ISEM) faulty';
   			        16777936:
   			            qLast_Diagnostics_String := 'F372 Sensor electronics (ISEM) faulty';
   			        16777937:
   			            qLast_Diagnostics_String := 'F373 Sensor electronics (ISEM) faulty';
   			        16778224:
   			            qLast_Diagnostics_String := 'F378 Electronic module supply voltage faulty';
   			        16778408:
   			            qLast_Diagnostics_String := 'F278 Display module defective';
   			        16778409:
   			            qLast_Diagnostics_String := 'F278 Display module defective';
   			        16778490:
   			            qLast_Diagnostics_String := 'F419 Power cycle required';
   			        16843466:
   			            qLast_Diagnostics_String := 'F331 Firmware update failed in module 2';
   			        16909002:
   			            qLast_Diagnostics_String := 'F331 Firmware update failed in module 3';
   			        33554576:
   			            qLast_Diagnostics_String := 'C484 Failure mode simulation active';
   			        33554579:
   			            qLast_Diagnostics_String := 'C485 Process variable simulation active';
   			        33554580:
   			            qLast_Diagnostics_String := 'C453 Flow override active';
   			        33554782:
   			            qLast_Diagnostics_String := 'C495 Diagnostic event simulation active';
   			        33554926:
   			            qLast_Diagnostics_String := 'C302 Device verification active';
   			        33554948:
   			            qLast_Diagnostics_String := 'C412 Processing download';
   			        67108970:
   			            qLast_Diagnostics_String := 'M438 Dataset different';
   			        67109090:
   			            qLast_Diagnostics_String := 'M311 Sensor electronics (ISEM) faulty';
   			        67109921:
   			            qLast_Diagnostics_String := 'M230 Date/time incorrect';
   			        67110029:
   			            qLast_Diagnostics_String := 'M231 Date/time not available';
   			        67110030:
   			            qLast_Diagnostics_String := 'M230 Date/time incorrect';
   			        134217873:
   			            qLast_Diagnostics_String := 'S842 Process value below limit';
   			        134217874:
   			            qLast_Diagnostics_String := 'S862 Partly filled pipe';
   			        134217921:
   			            qLast_Diagnostics_String := 'S833 Sensor electronics temperature too low';
   			        134217923:
   			            qLast_Diagnostics_String := 'S832 Sensor electronics temperature too high';
   			        134217924:
   			            qLast_Diagnostics_String := 'S912 Medium inhomogeneous';
   			        134217925:
   			            qLast_Diagnostics_String := 'S834 Process temperature too high';
   			        134217926:
   			            qLast_Diagnostics_String := 'S835 Process temperature too low';
   			        134217928:
   			            qLast_Diagnostics_String := 'S046 Sensor limit exceeded';
   			        134217930:
   			            qLast_Diagnostics_String := 'S046 Sensor limit exceeded';
   			        134217932:
   			            qLast_Diagnostics_String := 'S140 Sensor signal asymmetrical';
   			        134217933:
   			            qLast_Diagnostics_String := 'S913 Medium unsuitable';
   			        134217934:
   			            qLast_Diagnostics_String := 'S374 Sensor electronics (ISEM) faulty';
   			        134217951:
   			            qLast_Diagnostics_String := 'S912 Medium inhomogeneous';
   			        134218005:
   			            qLast_Diagnostics_String := 'S912 Medium inhomogeneous';
   			        134218082:
   			            qLast_Diagnostics_String := 'S912 Medium inhomogeneous';
   			        134218088:
   			            qLast_Diagnostics_String := 'S948 Oscillation damping too high';
   			        134218182:
   			            qLast_Diagnostics_String := 'S944 Monitoring failed';
   
   				else
   
   					qLast_Diagnostics_String := 'Error Code unknown';
   
   				end_case;
   
   				Trigger := FALSE;
   				DeviceData.OldState := DeviceData.State;
   				DeviceData.State := DeviceData.MaxState;
   				DeviceData.CommSuccess := FALSE;
   				DeviceData.AcyclicData[0] := 0;
   				DeviceData.NewState := TRUE;
   
   			elsif DeviceData.CommTimeOut then
   
   				temp_string1 := 'Error in step ';
   				Temp_DINT := DeviceData.State;
   				DTOS(Temp_DINT, temp_string2);
   				CONCAT(temp_string1, temp_string2, qAOI_Diagnostic_String);
   
   				DeviceData.OldState := DeviceData.State;
   				DeviceData.State := DeviceData.MaxState;    // Check State
   				DeviceData.CommTimeOut := FALSE;
   				DeviceData.AcyclicData[0] := 0;
   				DeviceData.NewState := TRUE;
   
   			end_if;
   
   		//*********************************
   		98: // End Step Trigger Guard
   		//*********************************
   
   			DeviceData.State := 0;
   			CommAOIBusy := 0;
   			DeviceAOISendRequest.[DeviceData.DevicePort] := 0;
   			ActiveComPort := 0;
   			ActiveAOI := 0;
   			DataToSend[0] := 0;
   			DataToSend[1] := 0;
   			DataToSend[2] := 0;
   			DataToSend[3] := 0;
   			DataToSend[4] := 0;
   			DataToSend[5] := 0;
    			DataToSend[6] := 0;
   			DataToSend[7] := 0;
   			DataToSend[8] := 0;
   			DataToSend[9] := 0;
   			DeviceData.StateDone := FALSE;
   			Skip := 0;
   			DeviceData.State := 0;
   			firstTimeDone := FALSE;
   			DeviceData.NewState := FALSE;
   			DeviceData.OldState := 0;
   			ActiveAOI := FALSE;
   
   			if SimActive then
   
   				SimActive := FALSE;
   				SimChanged := FALSE;
   
   			elsif TotActive then
   
   				TotActive := FALSE;
   				TotChanged := FALSE;
   
   			elsif CondStatusActive then
   
   				CondStatusActive := FALSE;
   				CondStatusChanged := FALSE;
   
   			elsif HeartbeatVerificationActive then
   
   				HeartbeatVerificationActive := FALSE;
   				HeartbeatVerificationChanged := FALSE;
   
   			end_if;
   
   	end_case;
   
   	end_if;
   
   	//*************************
   	// Execution Area
   	//*************************
   
   	if DeviceData.State > StateMin and DeviceData.State < DeviceData.MaxState then
   
   		DataToSend[2] := DeviceData.DevicePort;
   		DataToSend[3] := CMD_Index;
   		DataToSend[4] := CMD_Subindex;
   		DataToSend[5].0 := CMD_Rd;
   		DataToSend[5].1 := CMD_Wr;
   		DataToSend[5].8 := CMD_ByteLength.0;  // Bits for the Length of the Data
   		DataToSend[5].9 := CMD_ByteLength.1;
   		DataToSend[5].10 := CMD_ByteLength.2;
   		DataToSend[5].11 := CMD_ByteLength.3;
   		DataToSend[5].12 := CMD_ByteLength.4;
   		DataToSend[5].13 := CMD_ByteLength.5;
   		DataToSend[5].14 := CMD_ByteLength.6;
   		DataToSend[5].15 := CMD_ByteLength.7;
   		DataToSend[5].7 := Trigger;
   
   		qCommError := CommError;
   
   	end_if;
   
   end_if;
END_ROUTINE
END_ADD_ON_INSTRUCTION
